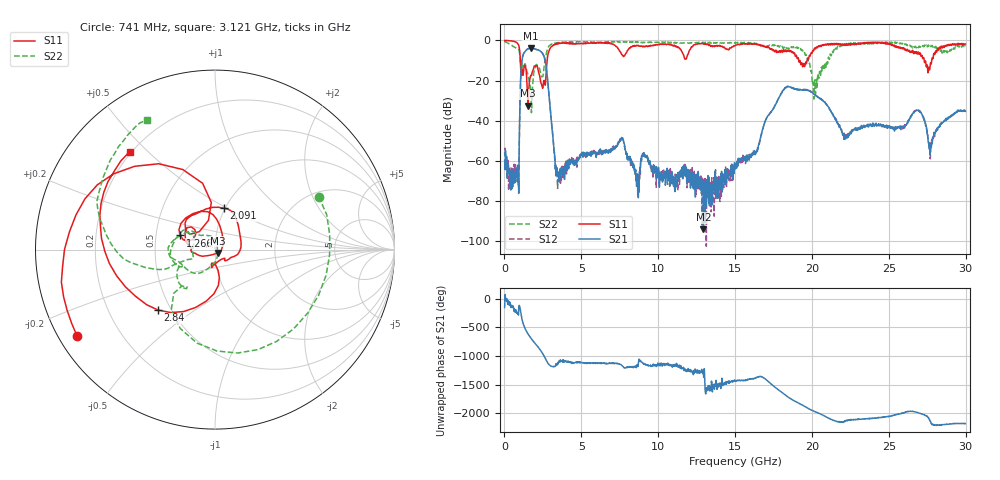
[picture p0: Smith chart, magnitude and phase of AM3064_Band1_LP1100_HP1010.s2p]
# Hz S DB R 50.0
!freq dBS11 angS11 dBS21 angS21 dBS12 angS12 dBS22 angS22
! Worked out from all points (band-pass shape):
!   1600 points, 10 MHz to 29.98 GHz, reference 50 ohm
!   highest |S21| = -3.89 dB at 1.716 GHz (marker M1); lowest = -94.0 dB at 12.94 GHz (marker M2)
!   |S21| within 3 dB of the highest: 1.23 GHz to 2.507 GHz (1.277 GHz wide, 68.3 % of centre)
!   lowest |S11| = -32.5 dB at 1.528 GHz (marker M3), VSWR 1.05, Z = 51.4 - j1.93 ohm
!   |S11| at or under -10 dB: 1.031 GHz to 2.775 GHz (1.744 GHz wide, 91.6 % of centre); 19.14 GHz to 19.68 GHz (541.8 MHz wide, 2.79 % of centre); 27.3 GHz to 27.79 GHz (488 MHz wide, 1.77 % of centre)
!   |S22| runs from -36.0 to -0.4 dB; largest |S21 - S12| = 0.0091
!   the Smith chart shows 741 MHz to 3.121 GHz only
!   S11 on the Smith chart (normalised r, x): 741 MHz: 0.05, -0.29; 1.266 GHz: 0.67, +0.11; 2.091 GHz: 0.98, +0.48; 2.84 GHz: 0.43, -0.36; 3.121 GHz: 0.19, +0.44
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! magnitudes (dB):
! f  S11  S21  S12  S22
! 10 MHz  0.0  -60.0  -55.7  -0.4
! 741 MHz  -0.8  -63.8  -67.8  -3.7
! 1.266 GHz  -13.5  -6.3  -6.3  -12.8
! 1.528 GHz  -32.5  -4.2  -4.2  -17.3
! 1.716 GHz  -17.4  -3.9  -3.9  -26.5
! 2.091 GHz  -12.6  -4.5  -4.6  -12.0
! 2.84 GHz  -6.7  -22.5  -22.4  -3.5
! 3.121 GHz  -2.8  -45.4  -45.7  -1.8
! 3.553 GHz  -1.4  -70.5  -69.9  -1.1
! 5.015 GHz  -1.4  -56.2  -56.9  -0.6
! 7.62 GHz  -7.0  -49.2  -48.3  -0.7
! 8.613 GHz  -2.6  -71.0  -66.3  -0.9
! 10 GHz  -2.1  -67.1  -65.6  -1.0
! 12.94 GHz  -1.7  -94.0  -69.1  -1.0
! 15 GHz  -2.5  -62.2  -63.0  -1.4
! 18.23 GHz  -5.5  -23.8  -23.9  -4.0
! 19.99 GHz  -6.5  -25.8  -25.9  -17.6
! 22.17 GHz  -2.4  -46.9  -47.4  -2.0
! 25 GHz  -1.5  -43.0  -42.8  -1.1
! 26.93 GHz  -5.8  -35.0  -34.8  -3.6
! 27.71 GHz  -11.3  -53.1  -56.7  -2.5
! 29.98 GHz  -1.8  -35.3  -35.1  -2.9
